
FUNCTION_BLOCK FB100

TITLE =   <Analog Input>
//
//   Este FB funciona con todas las tarjetas de entrada analogica con el
//   rango de 0 a 27648,
//
//

AUTHOR:   H3     //  max. 8 Zeichen / max. 8 characters
FAMILY:   ANALOG   //  max. 8 Zeichen / max. 8 characters
NAME:     AN_INP //  max. 8 Zeichen / max. 8 characters
VERSION:  01.01    //  max. 15.15
//KNOW_HOW_PROTECT

//  Parametros del FB
//  Entradas
//	PIW_ENT		WORD	Periferia de entrada
//  CONF		WORD	Palabra de configuracion 	Bit O 	Activar Valor Substituto
//    												Bit 1	Activar Alarma baja
//   												Bit 2	SPARE
//													Bit 3	Activar Alarma muy Baja
//													Bit 4 	SPARE
//													Bit 5	Activar Alarma Alto valor
//													Bit 6	SPARE
//													Bit 7	Activar Alarma muy Alto valor
//													Bit 8	SPARE
//													Bit 9 a Bit 15 Para uso futuro
//
//	VAL_SUST	REAL	Valor substituto
//	LIM_ING_SUP	REAL	Valor Superior de Ingenieria
//	LIM_ING_INF	REAL	Valor Inferiro de Ingenieria
//	LIMBAJO		REAL	Limie para alarma por bajo valor
//	LIMMUYBAJO	REAL	Limie para alarma por muy bajo valor
//	LIMALTO		REAL	Limite para alarma por alto valor
//	LIMMUYALTO	REAL	Limite para alarma por muy bajo valor
//
//	Salildas
//	VAL_SALIDA	REAL	Valor de salida escalado
//	AL_BAJO		BOOL	Alarma Activa por bajo valor
//	AL_MUYBAJO	BOOL	Alarma Activa por muy bajo valor
//	AL_ALTO		BOOL	Alarma Activa por Alto Valor
//	AL_MUYALTO	BOOL	Alarma por muy alto Valor
//	FALLA_SEN	BOOL	Alarma por falla de sensor o sensor fuera de rango
//	AL_PRESENT	BOOL	Esta en uno siempre que haya alguna alarma presente
//
VAR_INPUT
  PIW_ENT : WORD;
  CONF : WORD;
  VAL_SUST, LIM_ING_SUP, LIM_ING_INF, LIMBAJO, LIMMUYBAJO, LIMALTO, LIMMUYALTO : REAL;
  Indef : BOOL;
  TIEM_AL_ACTIVO, TIEM_AL_DESACT : TIME;
END_VAR

VAR_OUTPUT
  VAL_SALIDA : REAL;
  AL_BAJO, AL_MUYBAJO, AL_ALTO, AL_MUYALTO, FALLA_SEN, AL_PRESENT : BOOL;
END_VAR

VAR
  piw_real : REAL;
  TEMP1, TEMP3, TEMP5, TEMP7 : TON;
  TEMP2, TEMP4, TEMP6, TEMP8 : TOF;

END_VAR

VAR_TEMP
span : real;
pendiente : real;
TMP_TEMP1_IN, TMP_TEMP1_Q : BOOL;
TMP_TEMP1_ET : TIME;
TMP_TEMP2_IN, TMP_TEMP2_Q : BOOL;
TMP_TEMP2_ET : TIME;
TMP_TEMP3_IN, TMP_TEMP3_Q : BOOL;
TMP_TEMP3_ET : TIME;
TMP_TEMP4_IN, TMP_TEMP4_Q : BOOL;
TMP_TEMP4_ET : TIME;
TMP_TEMP5_IN, TMP_TEMP5_Q : BOOL;
TMP_TEMP5_ET : TIME;
TMP_TEMP6_IN, TMP_TEMP6_Q : BOOL;
TMP_TEMP6_ET : TIME;
TMP_TEMP7_IN, TMP_TEMP7_Q : BOOL;
TMP_TEMP7_ET : TIME;
TMP_TEMP8_IN, TMP_TEMP8_Q : BOOL;
TMP_TEMP8_ET : TIME;

END_VAR

BEGIN
NETWORK
TITLE =   <PALABRA DE CONFIGURACION>

		L #conf; 	// Carga la palabra de configuracion y se transfiere a una palabra local
		T lw 100;


NETWORK
TITLE =   <Calculo de el valor de salida con valores normalizados>
// Si esta el bit de valor subsituto val_salida = val_sust
		AN L 101.0;
		JC VCLC;
		L VAL_SUST;

		JU SAL;
// Val_salida = (((lim_ing_sup - lim_ing_inf) / 27648) * piw_ent) + lim_ing_inf;
VCLC:	l lim_ing_sup;
		l lim_ing_inf;
		-r;
		l 27648.0;
		/r;
		t pendiente;

  		l piw_ent;
  		itd;
  		dtr;
  		l pendiente;
  		*r;
  		l lim_ing_inf;
  		+r;
SAL:	t val_salida;



NETWORK
TITLE =   <Alarmas>
// ALARMA BAJO NIVEL

		L VAL_SALIDA;
		L LIMBAJO;
		<R;
		A L 101.1;						// BIT DE CONFIGURACION ACTIVACION DE ALARMA POR BAJO NIVEL ACTIVA
		= TMP_TEMP1_IN;


		CALL TEMP1 (                    // TIMER ON DELAY
		IN := TMP_TEMP1_IN,
		PT := TIEM_AL_ACTIVO,
		Q := TMP_TEMP1_Q,
		ET:= TMP_TEMP1_ET
		);

		A TMP_TEMP1_Q;
		= TMP_TEMP2_IN;

		CALL TEMP2 (					// TIMER OFF DELAY
		IN := TMP_TEMP2_IN,
		PT := TIEM_AL_DESACT,
		Q := TMP_TEMP2_Q,
		ET := TMP_TEMP2_ET
		);


		CLR;
		O TMP_TEMP1_Q;
		O TMP_TEMP2_Q;
		= AL_BAJO;



// ALARMA MUY BAJO NIVEL

		L VAL_SALIDA;
		L LIMMUYBAJO;
		<R;
		A L 101.3;						// BIT DE CONFIGURACION ACTIVACION DE ALARMA POR MUY BAJO NIVEL ACTIVA
		= TMP_TEMP3_IN;

		CALL TEMP3 (
		IN := TMP_TEMP3_IN,
		PT := TIEM_AL_ACTIVO,
		Q := TMP_TEMP3_Q,
		ET:= TMP_TEMP3_ET
		);

		A TMP_TEMP3_Q;
		= TMP_TEMP4_IN;

		CALL TEMP4 (
		IN := TMP_TEMP4_IN,
		PT := TIEM_AL_DESACT,
		Q := TMP_TEMP4_Q,
		ET := TMP_TEMP4_ET
		);


		CLR;
		O TMP_TEMP3_Q;
		O TMP_TEMP4_Q;
		= AL_MUYBAJO;


// ALARMA ALTO NIVEL

		L VAL_SALIDA;
		L LIMALTO;
		>R;
		A L 101.5;						// BIT DE CONFIGURACION ACTIVACION DE ALARMA POR ALTO NIVEL ACTIVA
		= TMP_TEMP5_IN;

		CALL TEMP5 (
		IN := TMP_TEMP5_IN,
		PT := TIEM_AL_ACTIVO,
		Q := TMP_TEMP5_Q,
		ET:= TMP_TEMP5_ET
		);

		A TMP_TEMP5_Q;
		= TMP_TEMP6_IN;

		CALL TEMP6 (
		IN := TMP_TEMP6_IN,
		PT := TIEM_AL_DESACT,
		Q := TMP_TEMP6_Q,
		ET := TMP_TEMP6_ET
		);


		CLR;
		O TMP_TEMP5_Q;
		O TMP_TEMP6_Q;
		= AL_ALTO;

// ALARMA MUY ALTO NIVEL

		L VAL_SALIDA;
		L LIMMUYALTO;
		>R;
		A L 101.7;						// BIT DE CONFIGURACION ACTIVACION DE ALARMA POR MUY ALTO NIVEL ACTIVA
		= TMP_TEMP7_IN;

		CALL TEMP7 (
		IN := TMP_TEMP7_IN,
		PT := TIEM_AL_ACTIVO,
		Q := TMP_TEMP7_Q,
		ET:= TMP_TEMP7_ET
		);

		A TMP_TEMP7_Q;
		= TMP_TEMP8_IN;

		CALL TEMP8 (
		IN := TMP_TEMP8_IN,
		PT := TIEM_AL_DESACT,
		Q := TMP_TEMP8_Q,
		ET := TMP_TEMP8_ET
		);


		CLR;
		O TMP_TEMP7_Q;
		O TMP_TEMP8_Q;
		= AL_MUYALTO;

NETWORK
TITLE =   <ALARMA PRESENTE>
		CLR;
		A FALLA_SEN;
		R AL_BAJO;
		R AL_MUYBAJO;
		R AL_ALTO;
		R AL_MUYALTO;


		CLR;
		O AL_BAJO;
		O AL_MUYBAJO;
		O AL_ALTO;
		O AL_MUYALTO;
		= AL_PRESENT;


NETWORK
TITLE =   <FALLA DE SENSOR>
		O(;
		L PIW_ENT;
		L -100;
		<I;
		);
		O(;
		L PIW_ENT;
		L 28000;
		>I;
		);
		= FALLA_SEN;

NETWORK
TITLE =   <FALLA TARJETA O FALLA DE ESCLVO ESTATUS INDEFINIDO>
		AN  Indef;
		JC END;
		R FALLA_SEN;
		R AL_BAJO;
		R AL_MUYBAJO;
		R AL_ALTO;
		R AL_MUYALTO;

		L 0;
		T val_salida;
END: 	NOP 0;

END_FUNCTION_BLOCK

FUNCTION_BLOCK FB101

TITLE =   <ENTRADA ANALOGICA TEMPERATURAS>
//
//   Este FB funciona con todas las tarjetas de entrada analogica con el
//   rango de entrada de lectura directa de temperatura en celsiusx10,
//
//

AUTHOR:   H3       //  max. 8 Zeichen / max. 8 characters
FAMILY:   ANALOG   //  max. 8 Zeichen / max. 8 characters
NAME:     AN_TMP   //  max. 8 Zeichen / max. 8 characters
VERSION:  01.01    //  max. 15.15
//KNOW_HOW_PROTECT

//  Parametros del FB
//  Entradas
//	PIW_ENT		WORD	Periferia de entrada
//  CONF		WORD	Palabra de configuracion 	Bit O 	Activar Valor Substituto
//    												Bit 1	Activar Alarma baja
//   												Bit 2	SPARE
//													Bit 3	Activar Alarma muy Baja
//													Bit 4 	SPARE
//													Bit 5	Activar Alarma Alto valor
//													Bit 6	SPARE
//													Bit 7	Activar Alarma muy Alto valor
//													Bit 8	SPARE
//													Bit 9   SPARE
//                                                  Bit 10 a Bit 15 Para uso futuro
//
//	VAL_SUST	REAL	Valor substituto en grados ºC
//	LIMBAJO		REAL	Limie para alarma por bajo valor en grados ºC
//	LIMMUYBAJO	REAL	Limie para alarma por muy bajo valor en grados ºC
//	LIMALTO		REAL	Limite para alarma por alto valor en grados ºC
//	LIMMUYALTO	REAL	Limite para alarma por muy bajo valor en grados ºC
//
//	Salidas
//	VAL_celsius	REAL	Valor de salida escalado en grados centigrados
//	VAL_Farenhe	REAL	Valor de salida escalado en grados farenheit
//	AL_BAJO		BOOL	Alarma Activa por bajo valor
//	AL_MUYBAJO	BOOL	Alarma Activa por muy bajo valor
//	AL_ALTO		BOOL	Alarma Activa por Alto Valor
//	AL_MUYALTO	BOOL	Alarma por muy alto Valor
//	FALLA_SEN	BOOL	Alarma por falla de sensor o sensor fuera de rango
//	AL_PRESENT	BOOL	Esta en uno siempre que haya alguna alarma presente
//

VAR_INPUT
  PIW_ENT : WORD;
  CONF : WORD;
  VAL_SUST, LIMBAJO, LIMMUYBAJO, LIMALTO, LIMMUYALTO : REAL;
  TIEM_AL_ACTIVO, TIEM_AL_DESACT : TIME;
  Val_comp : real;
  INDEF : BOOL;
END_VAR

VAR_OUTPUT
  VAL_celsius : REAL;
  VAL_farenheit : REAL;
  AL_BAJO, AL_MUYBAJO, AL_ALTO, AL_MUYALTO, FALLA_SEN, AL_PRESENT : BOOL;
END_VAR

VAR
  piw_real : REAL;
  TEMP1, TEMP3, TEMP5, TEMP7 : TON;
  TEMP2, TEMP4, TEMP6, TEMP8 : TOF;

END_VAR

VAR_TEMP
Farenheit : bool;
TMP_TEMP1_IN, TMP_TEMP1_Q : BOOL;
TMP_TEMP1_ET : TIME;
TMP_TEMP2_IN, TMP_TEMP2_Q : BOOL;
TMP_TEMP2_ET : TIME;
TMP_TEMP3_IN, TMP_TEMP3_Q : BOOL;
TMP_TEMP3_ET : TIME;
TMP_TEMP4_IN, TMP_TEMP4_Q : BOOL;
TMP_TEMP4_ET : TIME;
TMP_TEMP5_IN, TMP_TEMP5_Q : BOOL;
TMP_TEMP5_ET : TIME;
TMP_TEMP6_IN, TMP_TEMP6_Q : BOOL;
TMP_TEMP6_ET : TIME;
TMP_TEMP7_IN, TMP_TEMP7_Q : BOOL;
TMP_TEMP7_ET : TIME;
TMP_TEMP8_IN, TMP_TEMP8_Q : BOOL;
TMP_TEMP8_ET : TIME;

END_VAR

BEGIN
NETWORK
TITLE =   <PALABRA DE CONFIGURACION>

		L #conf; 	// Carga la palabra de configuracion y se transfiere a una palabra local
		T lw 100;


NETWORK
TITLE =   <Calculo de el valor de salida con valores normalizados>
// Si esta el bit de valor subsituto val_salida = val_sust
		AN L 101.0;
		JC VCLC;
		L VAL_SUST;
		T VAL_celsius;

		L 1.8;
  		*R;
  		L 32.0;
  		+R;
		T VAL_farenheit;



		JU SUS;
// en centigrados = Val_salida = Tem ºC x 0.1
// en farenheit = Val_salida = (Tem ºC x 0.1) X 1.8 + 32
VCLC:	l piw_ent;
		itd;
  		dtr;
  		l 0.1;
  		*R;
  		l Val_comp;
  		+r;
  		T VAL_celsius;

  		L 1.8;
  		*R;
  		L 32.0;
  		+R;
		T VAL_farenheit;

SUS:	NOP 0;


NETWORK
TITLE =   <Alarmas>
// ALARMA BAJO NIVEL

		L VAL_celsius;
		L LIMBAJO;
		<R;
		A L 101.1;						// BIT DE CONFIGURACION ACTIVACION DE ALARMA POR BAJO NIVEL ACTIVA
		= TMP_TEMP1_IN;


		CALL TEMP1 (                    // TIMER ON DELAY
		IN := TMP_TEMP1_IN,
		PT := TIEM_AL_ACTIVO,
		Q := TMP_TEMP1_Q,
		ET:= TMP_TEMP1_ET
		);

		A TMP_TEMP1_Q;
		= TMP_TEMP2_IN;

		CALL TEMP2 (					// TIMER OFF DELAY
		IN := TMP_TEMP2_IN,
		PT := TIEM_AL_DESACT,
		Q := TMP_TEMP2_Q,
		ET := TMP_TEMP2_ET
		);


		CLR;
		O TMP_TEMP1_Q;
		O TMP_TEMP2_Q;
		= AL_BAJO;



// ALARMA MUY BAJO NIVEL

		L VAL_celsius;
		L LIMMUYBAJO;
		<R;
		A L 101.3;						// BIT DE CONFIGURACION ACTIVACION DE ALARMA POR MUY BAJO NIVEL ACTIVA
		= TMP_TEMP3_IN;

		CALL TEMP3 (
		IN := TMP_TEMP3_IN,
		PT := TIEM_AL_ACTIVO,
		Q := TMP_TEMP3_Q,
		ET:= TMP_TEMP3_ET
		);

		A TMP_TEMP3_Q;
		= TMP_TEMP4_IN;

		CALL TEMP4 (
		IN := TMP_TEMP4_IN,
		PT := TIEM_AL_DESACT,
		Q := TMP_TEMP4_Q,
		ET := TMP_TEMP4_ET
		);


		CLR;
		O TMP_TEMP3_Q;
		O TMP_TEMP4_Q;
		= AL_MUYBAJO;


// ALARMA ALTO NIVEL

		L VAL_celsius;
		L LIMALTO;
		>R;
		A L 101.5;						// BIT DE CONFIGURACION ACTIVACION DE ALARMA POR ALTO NIVEL ACTIVA
		= TMP_TEMP5_IN;

		CALL TEMP5 (
		IN := TMP_TEMP5_IN,
		PT := TIEM_AL_ACTIVO,
		Q := TMP_TEMP5_Q,
		ET:= TMP_TEMP5_ET
		);

		A TMP_TEMP5_Q;
		= TMP_TEMP6_IN;

		CALL TEMP6 (
		IN := TMP_TEMP6_IN,
		PT := TIEM_AL_DESACT,
		Q := TMP_TEMP6_Q,
		ET := TMP_TEMP6_ET
		);


		CLR;
		O TMP_TEMP5_Q;
		O TMP_TEMP6_Q;
		= AL_ALTO;

// ALARMA MUY ALTO NIVEL

		L VAL_celsius;
		L LIMMUYALTO;
		>R;
		A L 101.7;						// BIT DE CONFIGURACION ACTIVACION DE ALARMA POR MUY ALTO NIVEL ACTIVA
		= TMP_TEMP7_IN;

		CALL TEMP7 (
		IN := TMP_TEMP7_IN,
		PT := TIEM_AL_ACTIVO,
		Q := TMP_TEMP7_Q,
		ET:= TMP_TEMP7_ET
		);

		A TMP_TEMP7_Q;
		= TMP_TEMP8_IN;

		CALL TEMP8 (
		IN := TMP_TEMP8_IN,
		PT := TIEM_AL_DESACT,
		Q := TMP_TEMP8_Q,
		ET := TMP_TEMP8_ET
		);


		CLR;
		O TMP_TEMP7_Q;
		O TMP_TEMP8_Q;
		= AL_MUYALTO;

NETWORK
TITLE =   <ALARMA PRESENTE>
		CLR;
		A FALLA_SEN;
		R AL_BAJO;
		R AL_MUYBAJO;
		R AL_ALTO;
		R AL_MUYALTO;


		CLR;
		O AL_BAJO;
		O AL_MUYBAJO;
		O AL_ALTO;
		O AL_MUYALTO;
		= AL_PRESENT;


NETWORK
TITLE =   <FALLA DE SENSOR>
		O(;
		L PIW_ENT;
		L -500;
		<I;
		);
		O(;
		L PIW_ENT;
		L 10000;
		>I;
		);
		= FALLA_SEN;

NETWORK
TITLE =   <FALLA DE TARJETA O FALLA DE ESCLAVO ESTADO INDEFINIDO>

		AN INDEF;
		JC END1;

		R FALLA_SEN;
		R AL_BAJO;
		R AL_MUYBAJO;
		R AL_ALTO;
		R AL_MUYALTO;

		L 0;
		T VAL_celsius;
  		T VAL_farenheit;

END1: 	NOP 0;

END_FUNCTION_BLOCK

